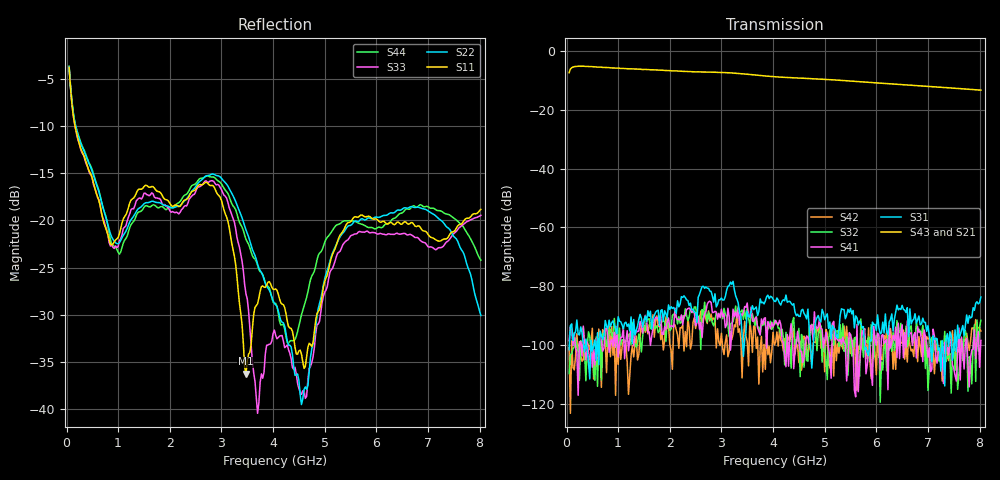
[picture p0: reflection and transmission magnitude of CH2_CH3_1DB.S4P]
!Agilent Technologies,E5071C,MY46316741,A.11.02
!Date: Thu May 28 14:39:09 2026
!Data & Calibration Information:
!1:CH2 INPUT 2:CH2 OUTPUT 3:CH3 INPUT 4:CH3 OUTPUT
!Freq	S11:SOLT4(ON)	S12:SOLT4(ON)	S13:SOLT4(ON)	S14:SOLT4(ON)
!	S21:SOLT4(ON)	S22:SOLT4(ON)	S23:SOLT4(ON)	S24:SOLT4(ON)
!	S31:SOLT4(ON)	S32:SOLT4(ON)	S33:SOLT4(ON)	S34:SOLT4(ON)
!	S41:SOLT4(ON)	S42:SOLT4(ON)	S43:SOLT4(ON)	S44:SOLT4(ON)
!PortZ  Port1:50+j0  Port2:50+j0  Port3:50+j0  Port4:50+j0
!Above PortZ is port z conversion or system Z0 setting when saving the data.
!When reading, reference impedance value at option line is always used.
# Hz S dB R 50
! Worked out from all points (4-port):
!   320 points, 50 MHz to 8.025 GHz, reference 50 ohm
!   strongest paths, dB at 50 MHz, 2.05 GHz, 4.05 GHz, 6.05 GHz, 8.025 GHz:
!     S43: -7.3, -6.7, -8.7, -10.9, -13.3
!     S21: -7.4, -6.8, -9.0, -11.1, -13.4
!     S31: -101.7, -87.6, -85.2, -94.2, -83.7
!     S41: -98.6, -93.6, -91.7, -96.6, -98.5
!     S32: -109.8, -90.0, -92.9, -97.4, -91.7
!     S42: -101.0, -108.3, -99.0, -104.4, -95.3
!   lowest |S11| = -36.2 dB at 3.475 GHz (marker M1), VSWR 1.03, Z = 48.7 - j0.768 ohm
!   |S11| at or under -10 dB: 164.8 MHz to end of sweep
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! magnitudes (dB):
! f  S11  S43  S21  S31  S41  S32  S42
! 50 MHz  -3.8  -7.3  -7.4  -101.7  -98.6  -109.8  -101.0
! 1.025 GHz  -21.4  -5.8  -6.0  -92.0  -99.6  -94.3  -98.1
! 2.85 GHz  -16.4  -7.2  -7.3  -85.5  -89.0  -93.5  -90.9
! 3.475 GHz  -36.2  -7.8  -8.0  -95.2  -87.2  -91.2  -97.1
! 4.55 GHz  -34.2  -9.2  -9.4  -88.2  -102.4  -96.5  -108.6
! 5.575 GHz  -19.6  -10.3  -10.5  -94.2  -115.4  -97.8  -97.8
! 8.025 GHz  -18.8  -13.3  -13.4  -83.7  -98.5  -91.7  -95.3
